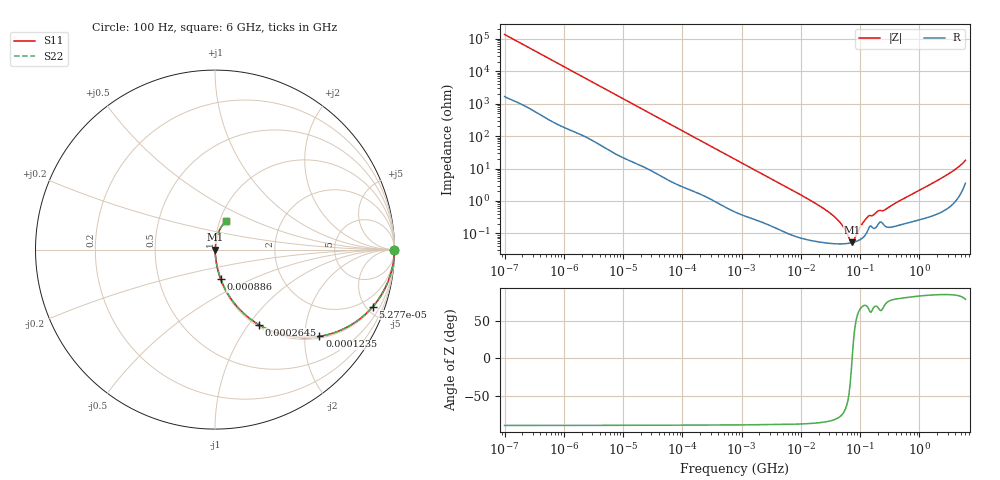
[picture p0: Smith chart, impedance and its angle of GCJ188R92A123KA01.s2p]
!Murata Part Number: GCJ188R92A123KA01
!These Parameters are Measured in Series Mode Connection
!Data Generated on Mar 13, 2026
!  o--ll--o
!Port1  Port2
!  o------o
!Operation Temp=25[degC], DC Bias Voltage=0[V]
!Freq. Start=100[Hz] Stop=6[GHz] 401[Steps]
# Hz S RI R 50
!Freq.(Hz) S11(Real) S11(Imag) S21(Real) S21(Imag) S12(Real) S12(Imag) S22(Real) S22(Imag)
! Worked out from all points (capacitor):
!   401 points, 100 Hz to 6 GHz, reference 50 ohm
!   read as one part in series: C = 11.6 nF near 109 Hz
!   lowest |Z| = 52.6 mohm at 74.56 MHz (marker M1)
!   series resonance near 73.53 MHz, so ESL is about 400 pH
!   S11 on the Smith chart (normalised r, x): 100 Hz: open; 52.77 kHz: 1.10, -5.50; 123.5 kHz: 1.05, -2.37; 264.5 kHz: 1.03, -1.12; 886 kHz: 1.01, -0.34; 6 GHz: 1.07, +0.35
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100  1 -0.000731  9.4e-06 0.000731  9.4e-06 0.000731  1 -0.000731
2008  0.9996 -0.0143  0.000425 0.0143  0.000425 0.0143  0.9996 -0.0143
12041  0.9916 -0.0836  0.00835 0.0836  0.00835 0.0836  0.9916 -0.0836
40335  0.924 -0.2563  0.076 0.2563  0.076 0.2563  0.924 -0.2563
52766  0.879 -0.3175  0.121 0.3175  0.121 0.3175  0.879 -0.3175
123542  0.5822 -0.4834  0.4178 0.4834  0.4178 0.4834  0.5822 -0.4834
264476  0.2434 -0.4179  0.7566 0.4179  0.7566 0.4179  0.2434 -0.4179
432798  0.1116 -0.3036  0.8884 0.3036  0.8884 0.3036  0.1116 -0.3036
774597  0.0403 -0.1851  0.9597 0.1851  0.9597 0.1851  0.0403 -0.1851
885955  0.0317 -0.1636  0.9683 0.1636  0.9683 0.1636  0.0317 -0.1636
2713602  0.00505 -0.056  0.995 0.056  0.995 0.056  0.00505 -0.056
1.555665e7  0.000684 -0.00966  0.9993 0.00966  0.9993 0.00966  0.000684 -0.00966
3.983537e7  0.000483 -0.00284  0.9995 0.00284  0.9995 0.00284  0.000483 -0.00284
5.211241e7  0.000478 -0.00154  0.9995 0.00154  0.9995 0.00154  0.000478 -0.00154
6.817316e7  0.000504 -0.000333  0.9995 0.000333  0.9995 0.000333  0.000504 -0.000333
7.455971e7  0.000522 6.21e-05  0.9995 -6.21e-05  0.9995 -6.21e-05  0.000522 6.21e-05
8.154455e7  0.000546 0.000461  0.9995 -0.000461  0.9995 -0.000461  0.000546 0.000461
1.066761e8  0.000691 0.00173  0.9993 -0.00173  0.9993 -0.00173  0.000691 0.00173
1.334425e8  0.00117 0.00297  0.9988 -0.00297  0.9988 -0.00297  0.00117 0.00297
3.124326e8  0.00157 0.00638  0.9984 -0.00638  0.9984 -0.00638  0.00157 0.00638
2.679998e9  0.00836 0.0569  0.9916 -0.0569  0.9916 -0.0569  0.00836 0.0569
6e9  0.0611 0.1591  0.9389 -0.1591  0.9389 -0.1591  0.0611 0.1591
